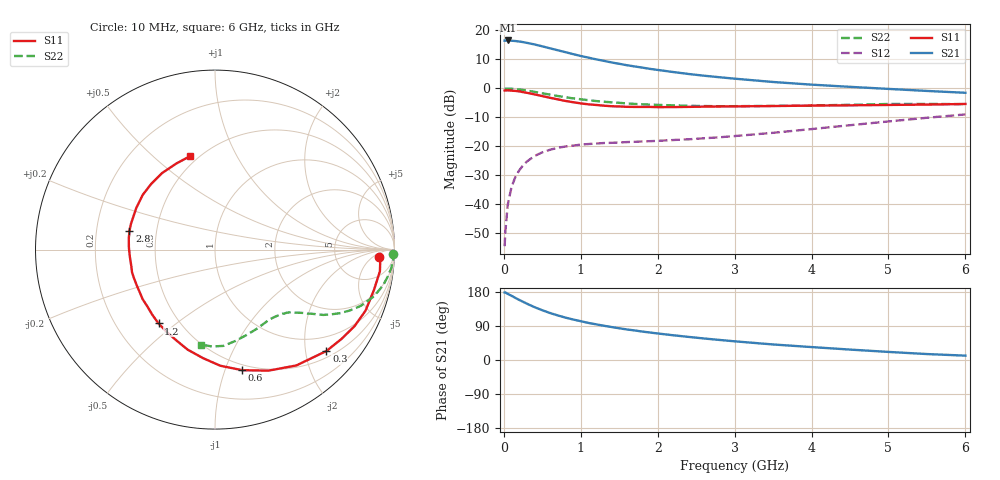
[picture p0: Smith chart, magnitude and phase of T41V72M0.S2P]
! Infineon Technologies  Discrete & RF Semiconductors
! BFR182T
! Si NPN RF Bipolar Junction Transistor in SC75
! VCE = 1.75 V  IC = 2 mA
! Common Emitter S-Parameters:  October  1999
# GHz  S  MA  R  50
!  f  S11  S21  S12  S22
! GHz  MAG  ANG  MAG  ANG  MAG  ANG  MAG  ANG
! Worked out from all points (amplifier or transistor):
!   36 points, 10 MHz to 6 GHz, reference 50 ohm
!   highest |S21| = 16.5 dB at 50 MHz (marker M1)
!   |S21| within 3 dB of that: start of sweep to 643.4 MHz
!   unconditionally stable (mu >= 1): 1.948 GHz to 4.388 GHz
!   at 250 MHz: K = 0.15, MSG = 21.3 dB, |S12| = -26.5 dB
!   at 1.4 GHz: K = 0.79, MSG = 13.9 dB, |S12| = -18.8 dB
!   at 6 GHz: K = 0.84, MSG = 3.7 dB, |S12| = -9.0 dB
!   lowest NFmin = 1.10 dB at 450 MHz
!   S11 on the Smith chart (normalised r, x): 10 MHz: 18, -9; 300 MHz: 0.64, -2.44; 600 MHz: 0.45, -1.15; 1.2 GHz: 0.39, -0.43; 2.8 GHz: 0.35, +0.09; 6 GHz: 0.45, +0.67
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0.01  0.9167 -2.6  6.678 178.3  0.0019 83.0  0.9899 -1.4
0.02  0.9224 -1.7  6.645 178.2  0.0034 91.4  0.987 -1.1
0.05  0.9267 -7.5  6.713 174.5  0.0097 89.2  0.994 -3.1
0.1  0.9137 -14.3  6.638 169.5  0.02 83.5  0.987 -6.1
0.15  0.9051 -22.1  6.565 163.8  0.0297 77.7  0.9735 -9.0
0.2  0.8867 -28.8  6.439 158.6  0.0386 75.0  0.9585 -11.8
0.3  0.8395 -42.3  6.104 148.6  0.0549 67.2  0.918 -16.8
0.4  0.7887 -54.9  5.728 139.3  0.0682 60.9  0.8707 -21.1
0.5  0.7372 -66.2  5.315 131.3  0.079 56.2  0.8243 -24.3
0.6  0.6886 -77.3  4.913 124.0  0.0874 52.2  0.7809 -27.0
0.8  0.608 -96.4  4.22 111.9  0.0994 45.9  0.7046 -31.1
0.9  0.5778 -105.3  3.899 106.9  0.1031 43.8  0.6728 -32.4
1.1  0.531 -120.7  3.394 97.8  0.1098 40.9  0.6259 -34.7
1.2  0.5181 -127.4  3.168 94.1  0.1117 40.2  0.6049 -35.7
1.4  0.4925 -139.8  2.803 87.0  0.1151 39.2  0.5759 -37.6
1.6  0.4811 -151.4  2.511 80.6  0.1187 39.5  0.5502 -39.3
2.2  0.4762 -175.4  1.917 65.3  0.1287 43.3  0.5103 -45.6
2.8  0.4879 167.7  1.559 53.0  0.1434 48.8  0.4929 -53.3
3.5  0.496 152.2  1.29 41.0  0.1714 54.3  0.4993 -62.7
4.5  0.5102 134.1  1.064 27.5  0.2318 57.6  0.5216 -77.4
5.5  0.5258 114.2  0.904 15.7  0.3115 55.4  0.5402 -91.8
6  0.5391 104.8  0.84 11.5  0.3557 52.5  0.5345 -98.3
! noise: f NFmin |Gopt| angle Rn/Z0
0.45  1.1  0.42  29  0.36
0.9  1.2  0.4  58  0.3
1.8  1.85  0.32  126  0.22
